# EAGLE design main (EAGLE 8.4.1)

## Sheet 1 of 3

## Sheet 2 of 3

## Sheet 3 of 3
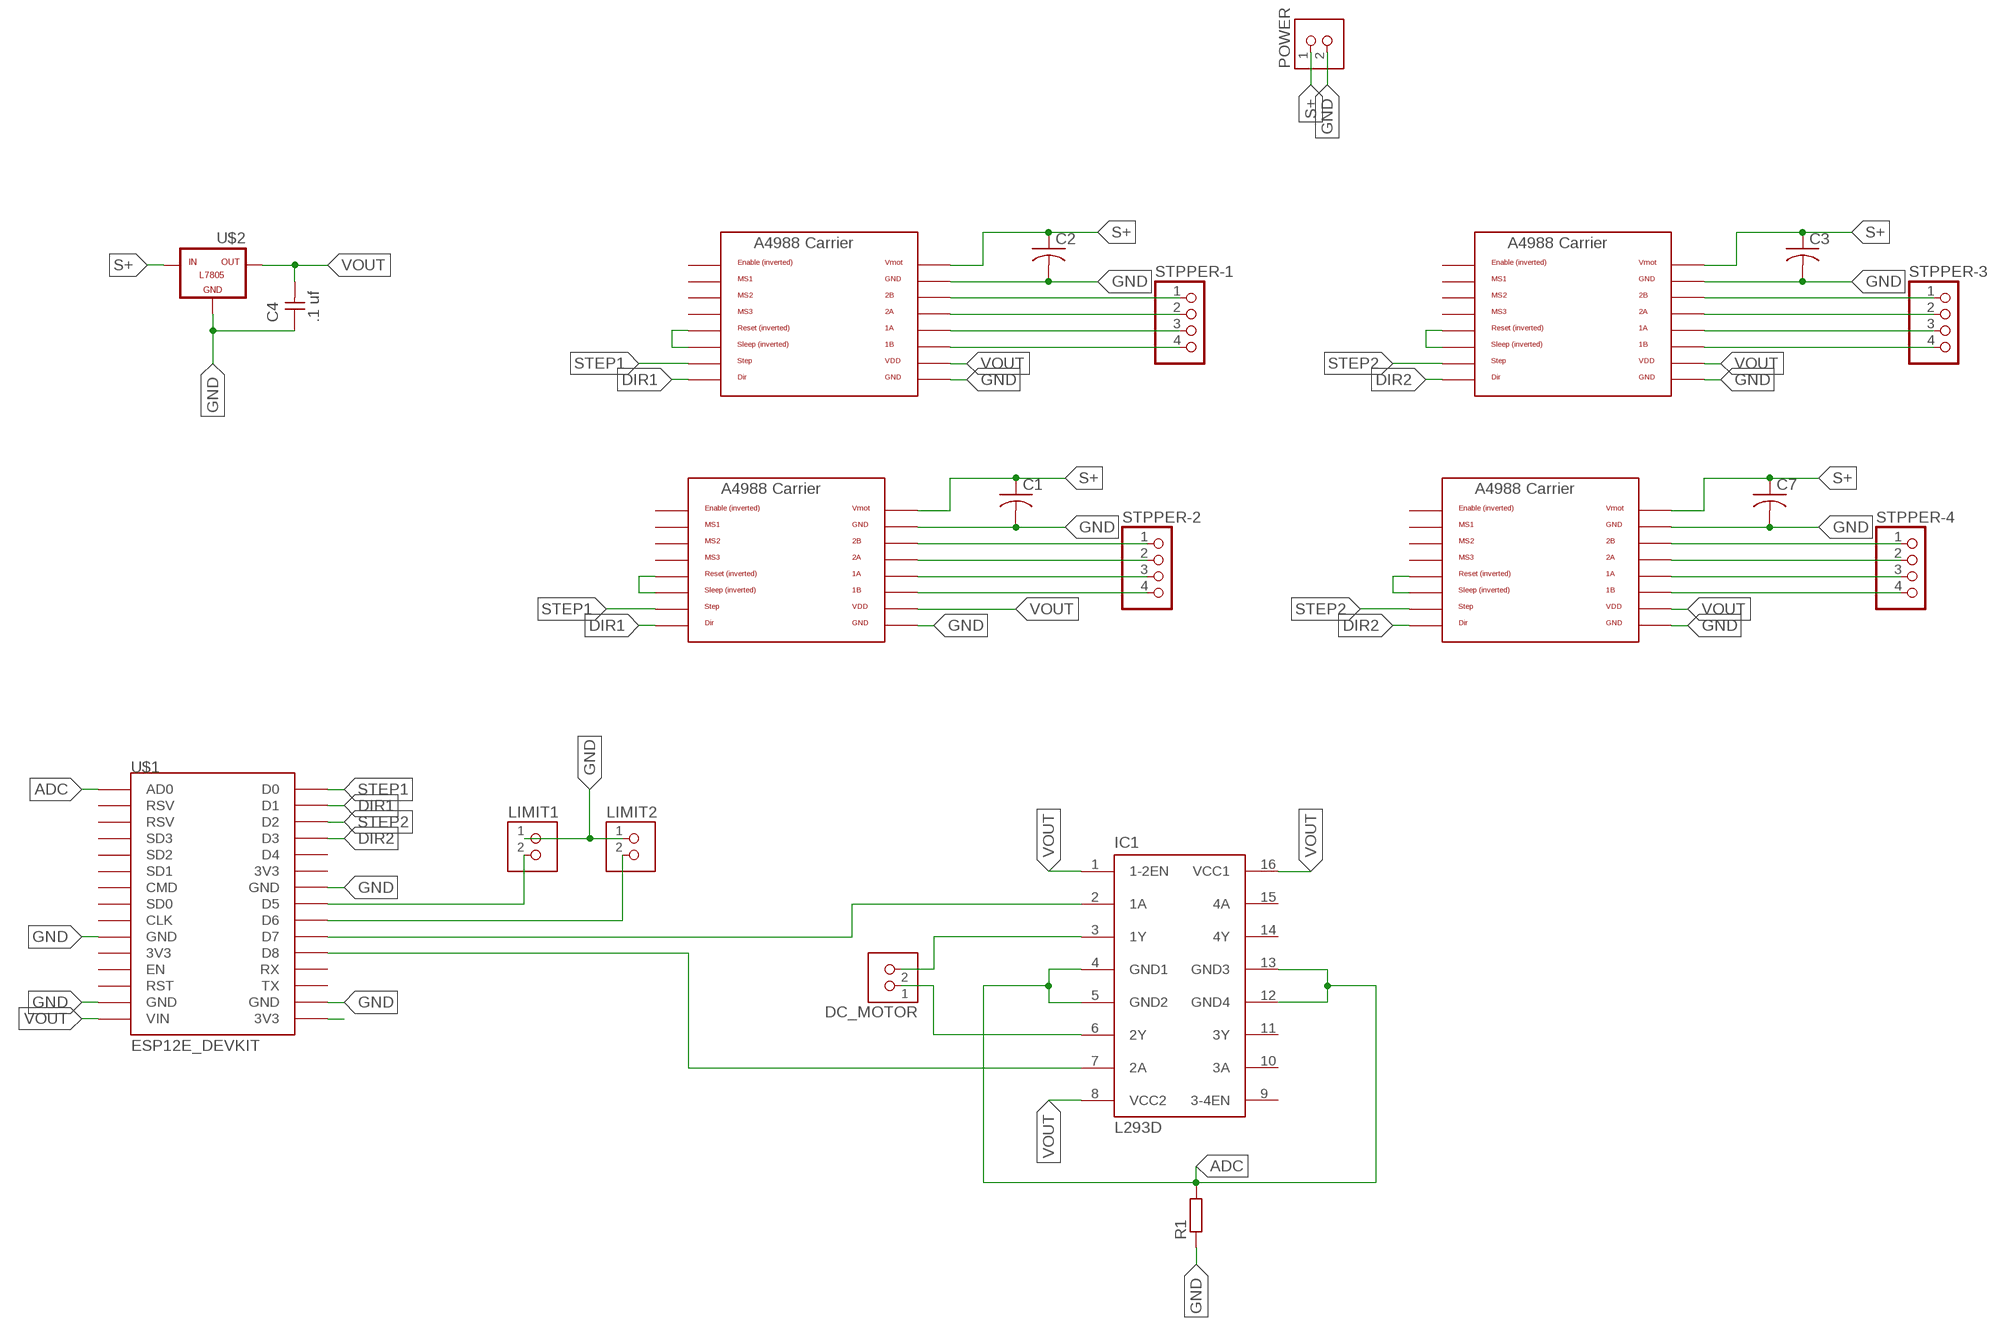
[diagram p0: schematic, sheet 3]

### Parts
A4988-01  A4988-1  POLOLU_A4983CARRIER  [A4988BREAKOUT]
A4988-02  A4988-1  POLOLU_A4983CARRIER  [A4988BREAKOUT]
A4988-03  A4988-1  POLOLU_A4983CARRIER  [A4988BREAKOUT]
A4988-04  A4988-1  POLOLU_A4983CARRIER  [A4988BREAKOUT]
C1  C-US050-024X044  [C050-024X044]
C2  C-US050-024X044  [C050-024X044]
C3  C-US050-024X044  [C050-024X044]
C4  .1 uf  CAP-UNPOLARIZEDFAB  [C1206FAB]
C7  C-US050-024X044  [C050-024X044]
DC_MOTOR  TERM-1X02-FABLAB  [ED555DS-2DS]
IC1  L293D  [DIL16]
LIMIT1  TERM-1X02-FABLAB  [ED555DS-2DS]
LIMIT2  TERM-1X02-FABLAB  [ED555DS-2DS]
POWER  TERM-1X02-FABLAB  [ED555DS-2DS]
R1  R-EU_0207/10  [0207/10]
STPPER-1  PINHD-1X4  [1X04]
STPPER-2  PINHD-1X4  [1X04]
STPPER-3  PINHD-1X4  [1X04]
STPPER-4  PINHD-1X4  [1X04]
U$1  ESP12E_DEVKIT  [ESP12E_DEVKIT]
U$2  -L7805  [L7805]

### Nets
ADC: IC1.4(GND1) IC1.5(GND2) IC1.12(GND4) IC1.13(GND3) R1.2 U$1.AD0
DIR1: A4988-01.DIR A4988-02.DIR U$1.D1
DIR2: A4988-03.DIR A4988-04.DIR U$1.D3
GND: A4988-01.GND A4988-01.GND@0(GND) A4988-02.GND A4988-02.GND@0(GND) A4988-03.GND A4988-03.GND@0(GND) A4988-04.GND A4988-04.GND@0(GND) C1.2 C2.2 C3.2 C4.1 C7.2 LIMIT1.1 LIMIT2.1 POWER.2 R1.1 U$1.GND@0(GND) U$1.GND@1(GND) U$1.GND@2(GND) U$1.GND@3(GND) U$2.GND
N$1: LIMIT1.2 U$1.D5
N$2: LIMIT2.2 U$1.D6
N$3: A4988-02.RST A4988-02.SLP(SLEEP)
N$6: DC_MOTOR.2 IC1.3(1Y)
N$7: DC_MOTOR.1 IC1.6(2Y)
N$8: A4988-01.RST A4988-01.SLP(SLEEP)
N$9: A4988-01.2B STPPER-1.1
N$10: A4988-01.2A STPPER-1.2
N$11: A4988-01.1A STPPER-1.3
N$12: A4988-01.1B STPPER-1.4
N$13: IC1.2(1A) U$1.D7
N$14: A4988-02.2B STPPER-2.1
N$15: A4988-02.2A STPPER-2.2
N$16: A4988-02.1A STPPER-2.3
N$17: A4988-02.1B STPPER-2.4
N$18: A4988-03.RST A4988-03.SLP(SLEEP)
N$19: A4988-03.2B STPPER-3.1
N$20: A4988-03.2A STPPER-3.2
N$21: A4988-03.1A STPPER-3.3
N$22: A4988-03.1B STPPER-3.4
N$23: A4988-04.RST A4988-04.SLP(SLEEP)
N$24: A4988-04.2B STPPER-4.1
N$25: A4988-04.2A STPPER-4.2
N$26: A4988-04.1A STPPER-4.3
N$27: A4988-04.1B STPPER-4.4
N$28: IC1.7(2A) U$1.D8
S+: A4988-01.VMOT A4988-02.VMOT A4988-03.VMOT A4988-04.VMOT C1.1 C2.1 C3.1 C7.1 POWER.1 U$2.IN
STEP1: A4988-01.STEP A4988-02.STEP U$1.D0
STEP2: A4988-03.STEP A4988-04.STEP U$1.D2
VCC: U$1.3V3@2(3V3)
VOUT: A4988-01.VDD A4988-02.VDD A4988-03.VDD A4988-04.VDD C4.2 IC1.1(1-2EN) IC1.8(VCC2) IC1.16(VCC1) U$1.VIN U$2.OUT
Unconnected: A4988-01.EN A4988-01.MS1 A4988-01.MS2 A4988-01.MS3 A4988-02.EN A4988-02.MS1 A4988-02.MS2 A4988-02.MS3 A4988-03.EN A4988-03.MS1 A4988-03.MS2 A4988-03.MS3 A4988-04.EN A4988-04.MS1 A4988-04.MS2 A4988-04.MS3 IC1.9(3-4EN) IC1.10(3A) IC1.11(3Y) IC1.14(4Y) IC1.15(4A) U$1.3V3@0(3V3) U$1.3V3@1(3V3) U$1.CLK U$1.CMD U$1.D4 U$1.EN U$1.RST U$1.RSV@0(RSV) U$1.RSV@1(RSV) U$1.RX U$1.SD0 U$1.SD1 U$1.SD2 U$1.SD3 U$1.TX

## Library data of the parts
A4988-01 = A4988_polu:POLOLU_A4983CARRIER; SPICEPREFIX: X
A4988-02-A4988-04 = A4988_polu:POLOLU_A4983CARRIER
C1-C3 C7 = rcl:C-US: CAPACITOR, American symbol
C4 = fab:CAP-UNPOLARIZED
DC_MOTOR LIMIT1 LIMIT2 POWER = fab:TERM-1X02: 3.5mm terminal block, 2 positions ED555-2DS as found in the fablab inventory.
IC1 = st-microelectronics:L293D: PUSH-PULL 4 CHANNEL DRIVER; MPN: L293D; OC_FARNELL: 9589619; OC_NEWARK: 56P8249
R1 = rcl:R-EU_: RESISTOR, European symbol
STPPER-1-STPPER-4 = pinhead:PINHD-1X4: PIN HEADER
U$1 = nodemcu:ESP12E_DEVKIT: ESP12E DEVKIT BOARD
U$2 = tango:-L7805

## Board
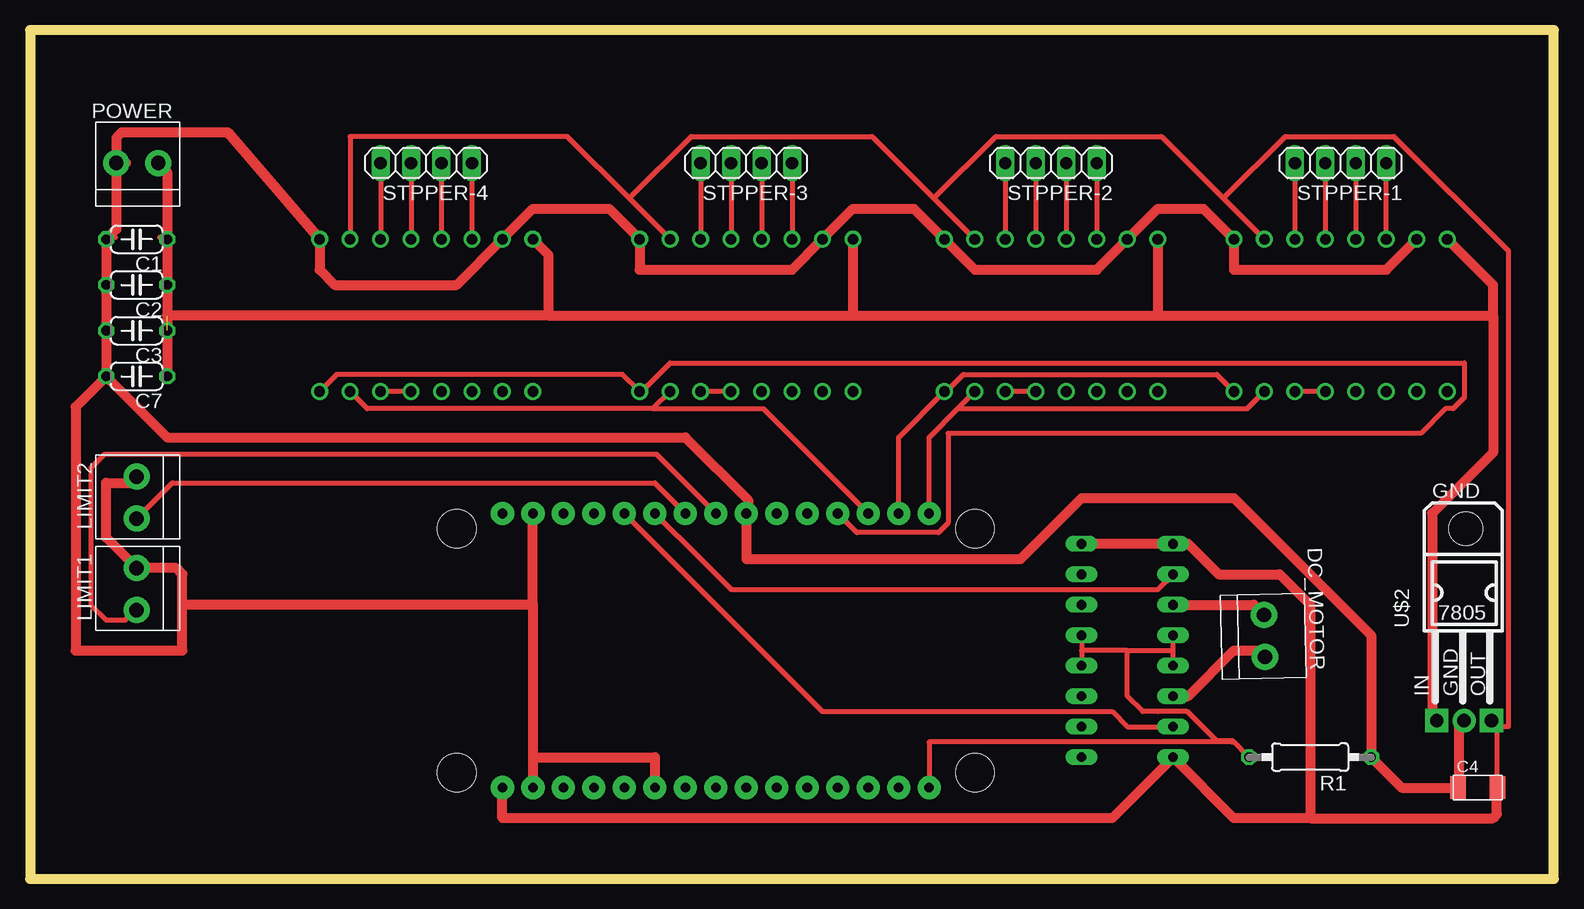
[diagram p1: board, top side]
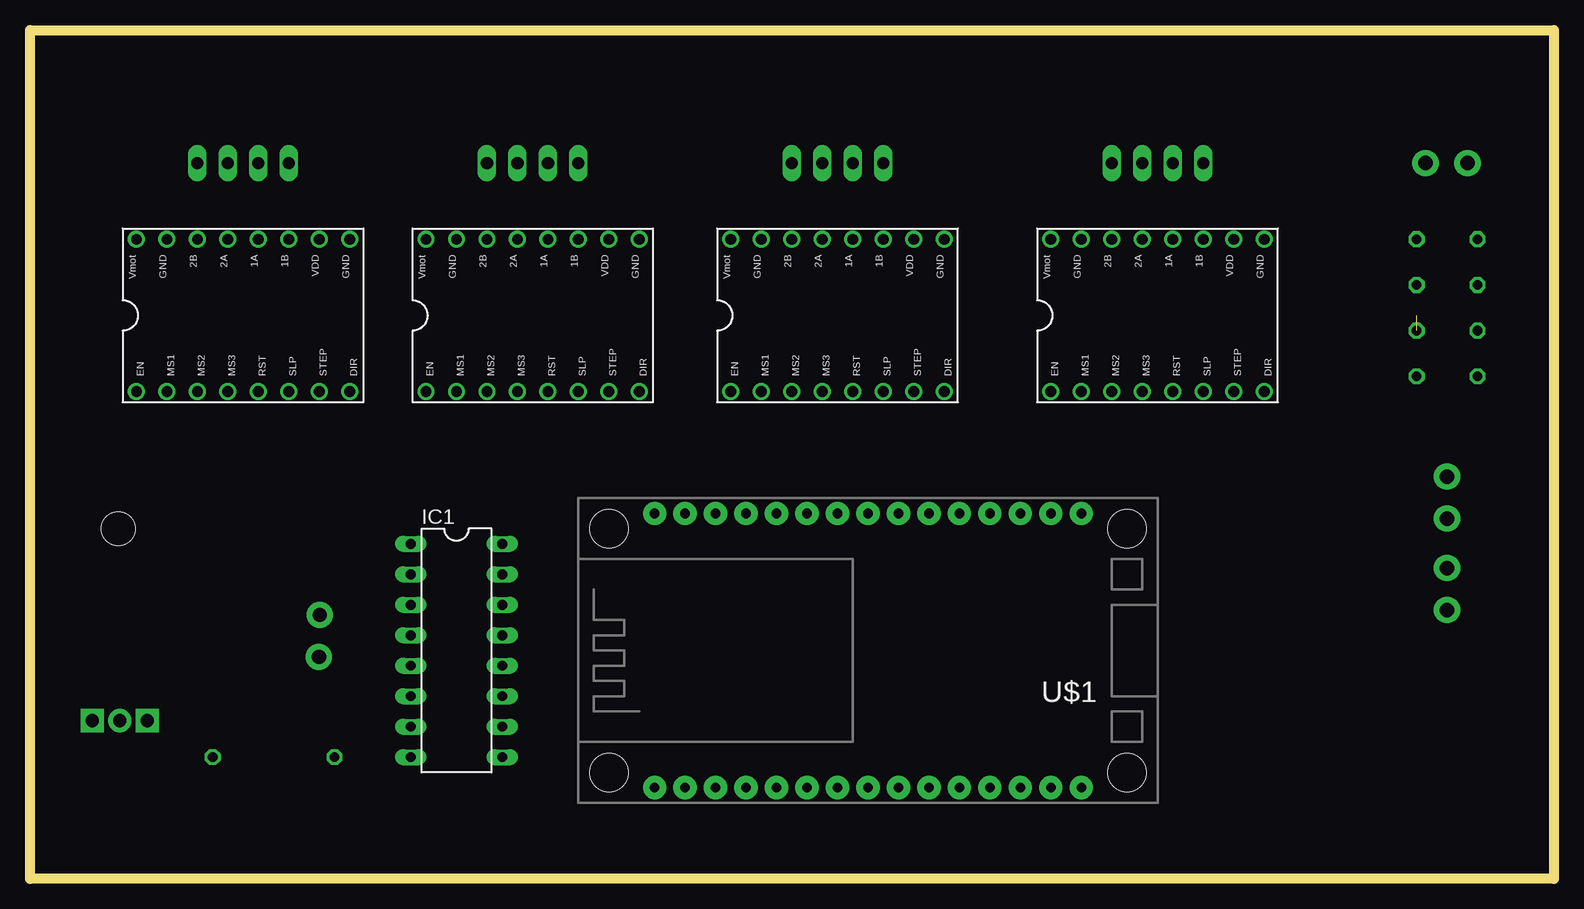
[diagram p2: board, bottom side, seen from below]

Size 126.98 x 70.79 mm. Coordinates in mm from the lower left corner, seen from the top.
Outline: 0,0 126.98,0 126.98,70.79 0,70.79 0,0
Copper layers (1*16): Top 0.035mm / dielectric 1.5mm / Bottom 0.035mm
Design rules "default *": minimum track width 16mil, minimum drill 0.35mm, track to track 16mil, track to pad 16mil, pad to pad 16mil, via to via 16mil, smd to smd 16mil, copper to edge 16mil, drill to drill 16mil, minimum pad ring 10mil, minimum via ring 8mil, stop-mask expansion 4mil, vias tented up to drill 0mil, thermal gap 10mil

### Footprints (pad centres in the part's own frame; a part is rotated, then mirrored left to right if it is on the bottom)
A4988BREAKOUT = drill 0.9: 1A 8.89,1.27; 1B 11.43,1.27; 2A 6.35,1.27; 2B 3.81,1.27; DIR 16.51,-11.43; EN -1.27,-11.43; GND 16.51,1.27; GND@0 1.27,1.27; MS1 1.27,-11.43; MS2 3.81,-11.43; MS3 6.35,-11.43; RST 8.89,-11.43; SLP 11.43,-11.43; STEP 13.97,-11.43; VDD 13.97,1.27; VMOT -1.27,1.27
C050-024X044 = drill 0.813 octagon: 1 -2.54,0; 2 2.54,0
C1206FAB = smd 1.27 x 1.905: 1 -1.651,0; 2 1.651,0
ED555DS-2DS = drill 1.2 pad 2.184: 1 1.8,0; 2 -1.7,0
DIL16 = drill 0.813 long: 1 -8.89,-3.81; 2 -6.35,-3.81; 3 -3.81,-3.81; 4 -1.27,-3.81; 5 1.27,-3.81; 6 3.81,-3.81; 7 6.35,-3.81; 8 8.89,-3.81; 9 8.89,3.81; 10 6.35,3.81; 11 3.81,3.81; 12 1.27,3.81; 13 -1.27,3.81; 14 -3.81,3.81; 15 -6.35,3.81; 16 -8.89,3.81
0207/10 = drill 0.813 octagon: 1 -5.08,0; 2 5.08,0
1X04 = drill 1.016 long: 1 -3.81,0; 2 -1.27,0; 3 1.27,0; 4 3.81,0
ESP12E_DEVKIT = drill 0.8 pad 1.93: 3V3@0 -11.43,-7.62; 3V3@1 11.43,5.08; 3V3@2 11.43,-17.78; AD0 -11.43,17.78; CLK -11.43,-2.54; CMD -11.43,2.54; D0 11.43,17.78; D1 11.43,15.24; D2 11.43,12.7; D3 11.43,10.16; D4 11.43,7.62; D5 11.43,0; D6 11.43,-2.54; D7 11.43,-5.08; D8 11.43,-7.62; EN -11.43,-10.16; GND@0 -11.43,-5.08; GND@1 -11.43,-15.24; GND@2 11.43,2.54; GND@3 11.43,-15.24; RST -11.43,-12.7; RSV@0 -11.43,15.24; RSV@1 -11.43,12.7; RX 11.43,-10.16; SD0 -11.43,0; SD1 -11.43,5.08; SD2 -11.43,7.62; SD3 -11.43,10.16; TX 11.43,-12.7; VIN -11.43,-17.78 | hole 3.2: -10.16,21.59; 10.16,21.59; 10.16,-21.59; -10.16,-21.59
L7805 = drill 1.1 pad 1.93: GND 0.127,-9.652 | drill 1.1 pad 1.93 square: IN -2.159,-9.652; OUT 2.413,-9.652 | hole 2.8: 0.254,6.35

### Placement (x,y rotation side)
A4988-01  116.84,52.07 0 bottom
A4988-02  92.71,52.07 0 bottom
A4988-03  67.31,52.07 0 bottom
A4988-04  40.64,52.07 0 bottom
C1  8.89,53.34 180 top
C2  8.89,49.53 180 top
C3  8.89,45.72 180 top
C4  120.65,7.62 0 top
C7  8.89,41.91 180 top
DC_MOTOR  102.87,20.32 271.3 top
IC1  91.44,19.05 270 bottom
LIMIT1  8.89,24.13 90 top
LIMIT2  8.89,31.75 90 top
POWER  8.89,59.69 0 top
R1  106.68,10.16 180 top
STPPER-1  109.22,59.69 180 top
STPPER-2  85.09,59.69 180 top
STPPER-3  59.69,59.69 180 top
STPPER-4  33.02,59.69 180 top
U$1  57.15,19.05 90 bottom
U$2  119.38,22.86 0 top

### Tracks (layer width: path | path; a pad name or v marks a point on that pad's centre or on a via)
ADC
  Top 0.406: IC1.13 87.63,19.05 | 87.63,19.05 IC1.12 | R1.2 100.25,11.51 | IC1.5 95.25,19.05 | 95.25,19.05 IC1.4 | 91.44,19.05 95.25,19.05 | 91.44,19.05 87.63,19.05 | U$1.AD0 74.93,11.43 100.17,11.43 100.25,11.51 | 100.25,11.51 98.9,11.51 96.44,13.97 93.98,13.97 92.71,13.97 91.44,15.24 91.44,19.05
DIR1
  Top 0.406: A4988-01.DIR 98.9,42.07 77.79,42.07 76.36,40.64 A4988-02.DIR 72.39,36.83 U$1.D1
DIR2
  Top 0.406: A4988-04.DIR 25.56,42.07 49.37,42.07 A4988-03.DIR 50.96,40.64 53.34,43.02 119.54,43.02 119.54,40.16 118.59,39.21 117.95,39.21 115.89,37.15 76.52,37.15 76.52,29.69 75.72,28.89 68.9,28.89 U$1.D3
GND
  Top 0.406: 100.49,53.34 A4988-01.GND | 39.53,53.34 A4988-04.GND@0 | 65.88,53.34 A4988-03.GND@0 | A4988-03.GND 50.96,53.34 | 91.28,53.34 A4988-02.GND@0 | 76.36,53.34 A4988-02.GND | 119.06,13.18 119.38,13.18 U$2.GND | 119.06,7.62 C4.1 | 7.14,53.5 6.35,53.5 C1.2 | 7.14,59.69 POWER.2 7.3,59.85 | 111.76,10.32 R1.1 | 59.85,30.48 U$1.GND@2 | 23.97,53.34 A4988-04.GND
  Top 0.813: POWER.2 8,59.69 | POWER.2 7.19,54.18 C1.2 C2.2 C3.2 C7.2 | 91.28,53.34 91.28,53.18 88.9,50.8 78.74,50.8 A4988-02.GND 73.66,55.88 68.58,55.88 A4988-03.GND@0 63.5,50.8 50.8,50.8 A4988-03.GND 48.26,55.88 41.91,55.88 A4988-04.GND@0 35.56,49.53 25.4,49.53 24.13,50.8 A4988-04.GND 16.51,62.23 7.62,62.23 7.19,61.8 POWER.2 | A4988-02.GND@0 93.98,55.88 97.79,55.88 A4988-01.GND 100.33,50.8 113.03,50.8 A4988-01.GND@0 | C7.2 3.81,39.37 3.81,19.05 12.7,19.05 12.7,22.86 | 12.7,22.86 12.7,25.4 12.17,25.93 LIMIT1.1 6.35,28.47 6.35,33.02 8.36,33.02 LIMIT2.1 | C7.2 6.51,41.91 | 41.91,22.86 12.7,22.86 | 41.91,22.86 41.91,10.16 | 41.91,10.16 U$1.GND@1 | 41.91,22.86 U$1.GND@3 | 41.91,10.16 52.07,10.16 U$1.GND@0 | 59.85,30.48 59.85,31.59 54.61,36.83 11.43,36.83 C7.2 | U$1.GND@2 59.69,26.67 82.55,26.67 87.63,31.75 100.33,31.75 111.76,20.32 R1.1 114.3,7.62 119.06,7.62 119.06,12.76 U$2.GND
N$1
  Top 0.406: U$1.D5 52.23,35.4 6.19,35.4 5.08,34.29 5.08,22.86 6.35,21.59 7.94,21.59 8.89,22.54 LIMIT1.2
N$2
  Top 0.406: 8.89,30.16 LIMIT2.2 11.86,33.02 52.07,33.02 U$1.D6
N$3
  Top 0.406: A4988-02.RST A4988-02.SLP
N$6
  Top 0.406: 102.23,22.54 102.71,22.07 DC_MOTOR.2
  Top 0.813: IC1.3 101.99,22.86 DC_MOTOR.2
N$7
  Top 0.813: IC1.6 96.52,15.24 100.33,19.05 102.38,19.05 DC_MOTOR.1
N$8
  Top 0.406: A4988-01.RST A4988-01.SLP
N$9
  Top 0.406: A4988-01.2B STPPER-1.1
N$10
  Top 0.406: STPPER-1.2 A4988-01.2A
N$11
  Top 0.406: STPPER-1.3 A4988-01.1A
N$12
  Top 0.406: STPPER-1.4 A4988-01.1B
N$13
  Top 0.406: U$1.D7 55.88,26.67 | 55.88,26.67 56.52,26.04 | 55.88,26.67 58.42,24.13 93.98,24.13 IC1.2
N$14
  Top 0.406: STPPER-2.1 A4988-02.2B
N$15
  Top 0.406: STPPER-2.2 A4988-02.2A
N$16
  Top 0.406: STPPER-2.3 A4988-02.1A
N$17
  Top 0.406: STPPER-2.4 A4988-02.1B
N$18
  Top 0.406: A4988-03.RST A4988-03.SLP
N$19
  Top 0.406: STPPER-3.1 A4988-03.2B
N$20
  Top 0.406: STPPER-3.2 A4988-03.2A
N$21
  Top 0.406: STPPER-3.3 A4988-03.1A
N$22
  Top 0.406: STPPER-3.4 A4988-03.1B
N$23
  Top 0.406: A4988-04.RST A4988-04.SLP
N$24
  Top 0.406: STPPER-4.1 A4988-04.2B
N$25
  Top 0.406: STPPER-4.2 A4988-04.2A
N$26
  Top 0.406: STPPER-4.3 A4988-04.1A
N$27
  Top 0.406: STPPER-4.4 A4988-04.1B
N$28
  Top 0.406: U$1.D8 66.04,13.97 90.17,13.97 91.44,12.7 IC1.7
S+  (1 unrouted)
  Top 0.406: 10.8,53.5 11.43,53.5 C1.1 | 10.8,59.69 POWER.1 | 93.82,53.34 A4988-02.VMOT
  Top 0.813: POWER.1 11.43,58.95 11.43,53.5 | C1.1 C2.1 C3.1 C7.1 | 121.92,46.99 121.92,49.53 A4988-01.VMOT | 121.92,46.99 121.92,35.56 116.84,30.48 116.84,13.97 117.73,13.08 117.35,13.08 | 117.35,13.08 U$2.IN 117.35,13.08 | 68.58,46.99 93.98,46.99 | 93.98,46.99 121.92,46.99 | A4988-03.VMOT 68.58,46.99 | A4988-02.VMOT 93.98,46.99 | 43.18,46.99 11.43,46.99 | 43.18,46.99 68.58,46.99 | A4988-04.VMOT 43.18,52.07 43.18,46.99
STEP1
  Top 0.406: 77.39,39.29 74.93,36.83 U$1.D0 | 77.39,39.29 A4988-02.STEP | A4988-01.STEP 101.44,39.21 77.47,39.21 77.39,39.29
STEP2
  Top 0.406: A4988-04.STEP 28.1,39.21 51.91,39.21 | A4988-03.STEP 51.91,39.21 | U$1.D2 61.12,39.21 51.91,39.21
VOUT
  Top 0.406: A4988-04.VDD 26.67,61.91 44.77,61.91 49.93,56.75 | A4988-03.VDD 49.93,56.75 | 75.33,56.75 70.17,61.91 55.09,61.91 49.93,56.75 | 75.33,56.75 A4988-02.VDD | 99.46,56.75 94.3,61.91 80.49,61.91 75.33,56.75 | 99.46,56.75 A4988-01.VDD | 122.24,13.18 122.24,7.62 | 121.92,13.18 U$2.OUT 121.76,13.34 | 122.08,7.62 122.24,7.62 | 122.24,7.62 C4.2 | 95.09,10.16 IC1.8 | 95.41,27.94 IC1.1 96.52,27.94 | 99.46,56.75 104.62,61.91 113.67,61.91 123.19,52.39 123.19,12.7 121.92,12.7 121.76,12.86
  Top 0.813: IC1.16 96.52,27.94 99.06,25.4 104.14,25.4 106.68,22.86 106.68,5.08 | 106.68,5.08 100.33,5.08 IC1.8 90.17,5.08 39.37,5.08 U$1.VIN | 106.68,5.08 121.92,5.08 122.24,5.4 122.24,7.62 | 122.24,13.18 121.83,13.18 U$2.OUT 121.79,12.89 121.76,12.86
